(* Logix 5000 AddOnInstructionDefinition export Banner_VSM_PD_v4; software revision 33.00 *)

TYPE Banner_VSM_PDI_v4 :   // UDT that records the converted prcoess data.
STRUCT
   Stability_Alarm : SINT;
   Detection_State : SINT;
END_STRUCT
END_TYPE

ADD_ON_INSTRUCTION Banner_VSM_PD_v4   (* revision 4.0, vendor Banner Engineering *)
// Takes the raw SINT information and converts that data into actual information.
VAR_IN_OUT
   SINT0 : SINT; {required}
   PROCESS_DATA : Banner_VSM_PDI_v4; {required}
END_VAR

ROUTINE Logic   (* ladder *)
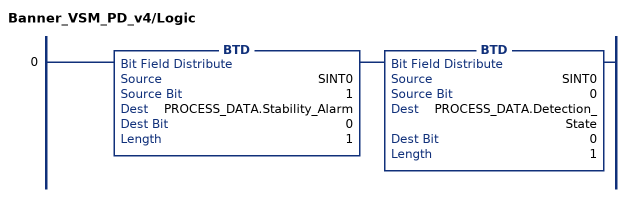
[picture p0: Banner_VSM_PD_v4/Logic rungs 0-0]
   0: BTD(SINT0,1,PROCESS_DATA.Stability_Alarm,0,1)BTD(SINT0,0,PROCESS_DATA.Detection_State,0,1);
END_ROUTINE
END_ADD_ON_INSTRUCTION
